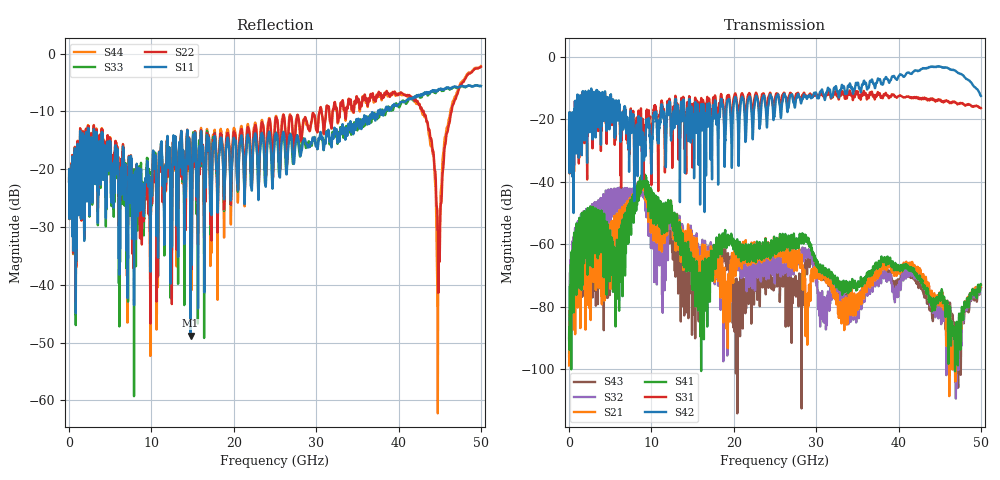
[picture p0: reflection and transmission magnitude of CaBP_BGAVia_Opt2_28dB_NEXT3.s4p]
!* Samtec Inc. NovaRay Examax Flyover System  *
!*  REV DATE  = 08/08/18  *
!*  TYPE  = TOUCHSTONE  *
!*  PORTS  = 4 port  *
!*  UNITS  = GHz  *
!*  DATA RANGE = DC  to 50 GHz; 10 MHz Step  *
!*  PARAMETER  = S  *
!*  FORMAT  = Real-Imaginary  *
!*  REFERENCE  = 50 ohms  *
!*  SOURCE  = HFSS  *
!*  VALIDATED  = No  *
!*  MANUFACTURER = SAMTEC  *
!*  INTERCONNECT = NVAx to EBCx to EBCx to NVAx  *
!*  [Full Channel NVAx to EBCx to EBCx to NVAx  with PCB Trace and BGA Via]  *
!*  BOUNDARY A  = Silicon BGA Ball Pad  *
!*  BOUNDARY B  = Silicon BGA Ball Pad  *
!*  NVAx (end a) ->>- (end b) NVAx  *
!*  Port 01 ->>- Port 02  *
!*  Port 03 ->>- Port 04  *
!***************************** CHANNEL MODEL ******************************************
# GHz S RI R 50
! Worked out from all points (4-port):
!   5000 points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, 10 MHz to 50 GHz, reference 50 ohm
!   strongest paths, dB at 10 MHz, 12.51 GHz, 25.01 GHz, 37.51 GHz, 50 GHz:
!     S42: -23.1, -21.4, -16.6, -6.9, -12.5
!     S31: -23.1, -28.5, -13.0, -11.3, -16.4
!     S41: -90.1, -51.8, -60.6, -66.8, -72.9
!     S21: -98.8, -51.3, -61.9, -69.9, -73.0
!     S32: -90.6, -51.4, -67.5, -71.9, -73.7
!     S43: -95.9, -61.2, -68.9, -68.8, -73.7
!   lowest |S11| = -48.8 dB at 14.75 GHz (marker M1), VSWR 1.01, Z = 49.7 - j0.221 ohm
!   |S11| at or under -10 dB: start of sweep to 37.51 GHz; 37.83997 GHz to 38.00552 GHz (165.6 MHz wide, 0.437 % of centre); 38.04261 GHz to 38.22467 GHz (182.1 MHz wide, 0.477 % of centre)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
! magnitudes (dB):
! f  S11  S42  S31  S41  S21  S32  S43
! 10 MHz  -22.1  -23.1  -23.1  -90.1  -98.8  -90.6  -95.9
! 8.94 GHz  -22.9  -25.6  -20.4  -37.3  -38.9  -42.3  -38.1
! 14.75 GHz  -48.8  -22.5  -22.0  -62.8  -55.8  -54.4  -65.8
! 18.97 GHz  -19.7  -26.7  -18.7  -55.6  -72.3  -76.9  -60.7
! 40.76 GHz  -8.3  -6.1  -12.9  -67.0  -66.7  -68.0  -69.6
! 44.81 GHz  -6.3  -3.1  -13.6  -78.4  -79.2  -83.4  -80.4
! 50 GHz  -5.6  -12.5  -16.4  -72.9  -73.0  -73.7  -73.7
